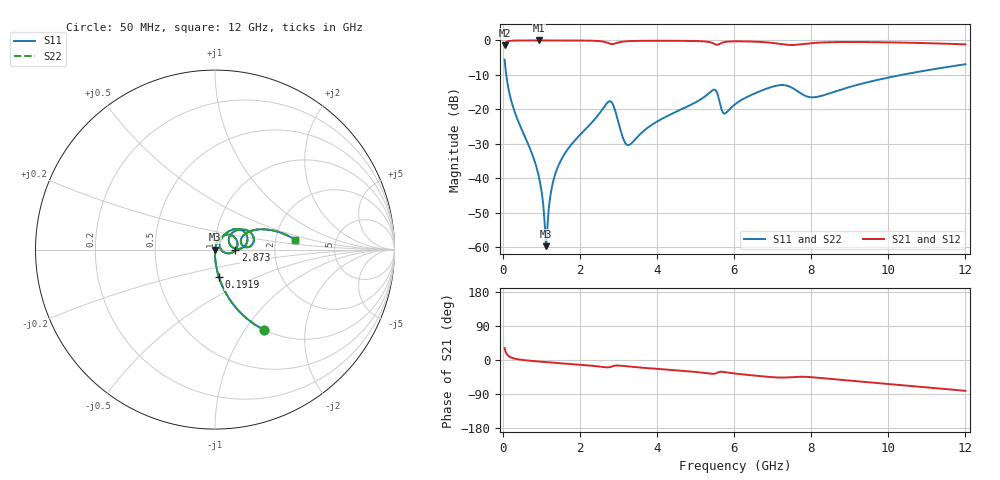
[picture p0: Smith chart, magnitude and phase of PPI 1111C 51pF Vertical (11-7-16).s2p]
# GHz S MA R 50
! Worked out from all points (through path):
!   1601 points, 50 MHz to 12 GHz, reference 50 ohm
!   highest |S21| = -0.01 dB at 946.2 MHz (marker M1); lowest = -1.4 dB at 50 MHz (marker M2)
!   group delay of S21, straight-line fit = 18.6 ps
!   lowest |S11| = -59.6 dB at 1.125 GHz (marker M3), VSWR 1.00, Z = 50.1 - j0.0185 ohm
!   |S11| at or under -10 dB: 92.51 MHz to 10.34 GHz (10.25 GHz wide, 196 % of centre)
!   |S22| runs from -59.6 to -5.6 dB; largest |S21 - S12| = 0
!   S11 on the Smith chart (normalised r, x): 50 MHz: 1.00, -1.24; 191.9 MHz: 1.00, -0.31; 2.873 GHz: 1.26, -0.01; 12 GHz: 2.59, +0.35
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0.05  0.5265 -58.5  0.8499 31.5  0.8499 31.5  0.5265 -58.5
0.1919063  0.1553 -81.8  0.9874 8.0  0.9874 8.0  0.1553 -81.8
0.94625  0.0101 -88.8  0.999 -4.1  0.999 -4.1  0.0101 -88.8
1.020938  0.005793 -85.0  0.9989 -4.7  0.9989 -4.7  0.005793 -85.0
1.088156  0.002281 -68.8  0.9989 -5.3  0.9989 -5.3  0.002281 -68.8
1.1255  0.001044 -10.2  0.9989 -5.6  0.9989 -5.6  0.001044 -10.2
1.162844  0.002113 53.9  0.9989 -5.9  0.9989 -5.9  0.002113 53.9
1.274875  0.007417 74.4  0.9988 -6.7  0.9988 -6.7  0.007417 74.4
1.409312  0.0137 77.0  0.9986 -7.8  0.9986 -7.8  0.0137 77.0
2.044156  0.04511 73.4  0.9958 -12.7  0.9958 -12.7  0.04511 73.4
2.723813  0.1268 35.4  0.9214 -19.4  0.9214 -19.4  0.1268 35.4
2.873187  0.1132 -1.4  0.8897 -15.8  0.8897 -15.8  0.1132 -1.4
3.119656  0.03858 -8.1  0.9616 -15.7  0.9616 -15.7  0.03858 -8.1
3.239156  0.03045 17.0  0.9744 -16.9  0.9744 -16.9  0.03045 17.0
4.038312  0.06851 59.1  0.9889 -23.7  0.9889 -23.7  0.06851 59.1
5.464844  0.1925 28.7  0.9038 -36.6  0.9038 -36.6  0.1925 28.7
5.741187  0.08743 20.6  0.9439 -31.8  0.9439 -31.8  0.08743 20.6
6.025  0.1186 43.7  0.9712 -35.8  0.9712 -35.8  0.1186 43.7
7.182656  0.2246 21.4  0.8928 -46.4  0.8928 -46.4  0.2246 21.4
8.019156  0.1499 13.9  0.9148 -45.5  0.9148 -45.5  0.1499 13.9
10.01331  0.2904 22.9  0.9379 -63.4  0.9379 -63.4  0.2904 22.9
12  0.4516 6.8  0.8771 -81.4  0.8771 -81.4  0.4516 6.8
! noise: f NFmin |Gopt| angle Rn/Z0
0.05  0.0003719  0.8662  0.6158  0.0005973
1.372  0.004011  0.6917  6.756  0.002525
2.701  0.04101  0.9327  13.31  0.1339
4.031  0.01793  0.7903  19.64  0.01712
5.36  0.04476  0.8845  25.95  0.07988
6.682  0.04387  0.8584  31.98  0.06127
8.012  0.07579  0.902  37.98  0.1515
9.341  0.04394  0.8173  43.45  0.04349
10.67  0.03918  0.7784  48.56  0.03018
12  0.03959  0.7643  53.43  0.02735
